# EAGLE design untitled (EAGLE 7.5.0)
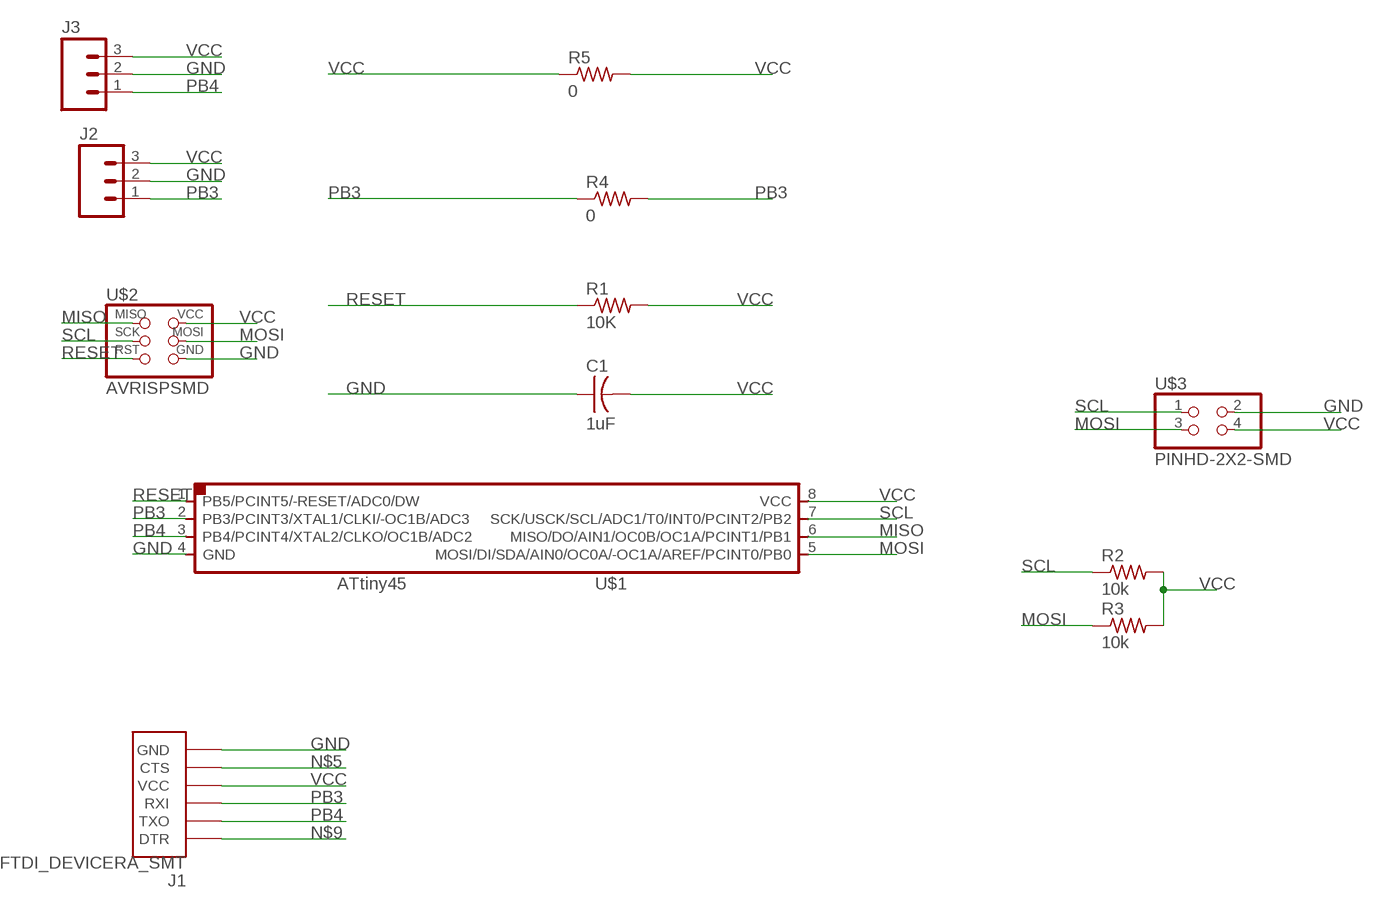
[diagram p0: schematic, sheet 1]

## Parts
C1  1uF  CAP-US1206  [C1206]
J1  FTDI_DEVICERA_SMT  [FTDI_DEVICE_RA_SMT]
J2  M03SMD_RA_MALE  [1X03_SMD_RA_MALE]
J3  M03SMD_RA_MALE  [1X03_SMD_RA_MALE]
R1  10K  RES-US1206FAB  [R1206FAB]
R2  10k  RES-US1206FAB  [R1206FAB]
R3  10k  RES-US1206FAB  [R1206FAB]
R4  0  RES-US1206FAB  [R1206FAB]
R5  0  RES-US1206FAB  [R1206FAB]
U$1  ATTINY45SI  [SOIC8]
U$2  AVRISPSMD  [2X03SMD]
U$3  PINHD-2X2-SMD  [2X02SMD]

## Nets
GND: C1.1 J1.6(GND) J2.2 J3.2 U$1.4(GND) U$2.6(GND) U$3.2
MISO: U$1.6(MISO/DO/AIN1/OC0B/OC1A/PCINT1/PB1) U$2.1(MISO)
MOSI: R3.1 U$1.5(MOSI/DI/SDA/AIN0/OC0A/-OC1A/AREF/PCINT0/PB0) U$2.4(MOSI) U$3.3
N$5: J1.5(CTS)
N$9: J1.1(DTR)
PB3: J1.3(RXI) J2.1 R4.1 R4.2 U$1.2(PB3/PCINT3/XTAL1/CLKI/-OC1B/ADC3)
PB4: J1.2(TXO) J3.1 U$1.3(PB4/PCINT4/XTAL2/CLKO/OC1B/ADC2)
RESET: R1.1 U$1.1(PB5/PCINT5/-RESET/ADC0/DW) U$2.5(RST)
SCL: R2.1 U$1.7(SCK/USCK/SCL/ADC1/T0/INT0/PCINT2/PB2) U$2.3(SCK) U$3.1
VCC: C1.2 J1.4(VCC) J2.3 J3.3 R1.2 R2.2 R3.2 R5.1 R5.2 U$1.8(VCC) U$2.2(VCC) U$3.4

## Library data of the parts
C1 = fab:CAP-US
J1 = SparkFun-Connectors:FTDI_DEVICE: Connector which mates to FTDI basic or FTDI cable.; PROD_ID: CONN-08971
J2 J3 = SparkFun-Connectors:M03: Header 3 Standard 3-pin 0.1" header. Use with straight break away headers (SKU : PRT-00116), right angle break away headers (PRT-00553), swiss pins (PRT-00743), machine pins (PRT-00117), and female headers (PRT-00115). Molex polarized connector foot print use with SKU : PRT-08232 with associated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; PROD_ID: CONN-10925
R1-R5 = fab:RES-US: Resistor (US Symbol)
U$1 = fab:ATTINY45
U$2 = fab:AVRISP
U$3 = fab:PINHD-2X2-SMD

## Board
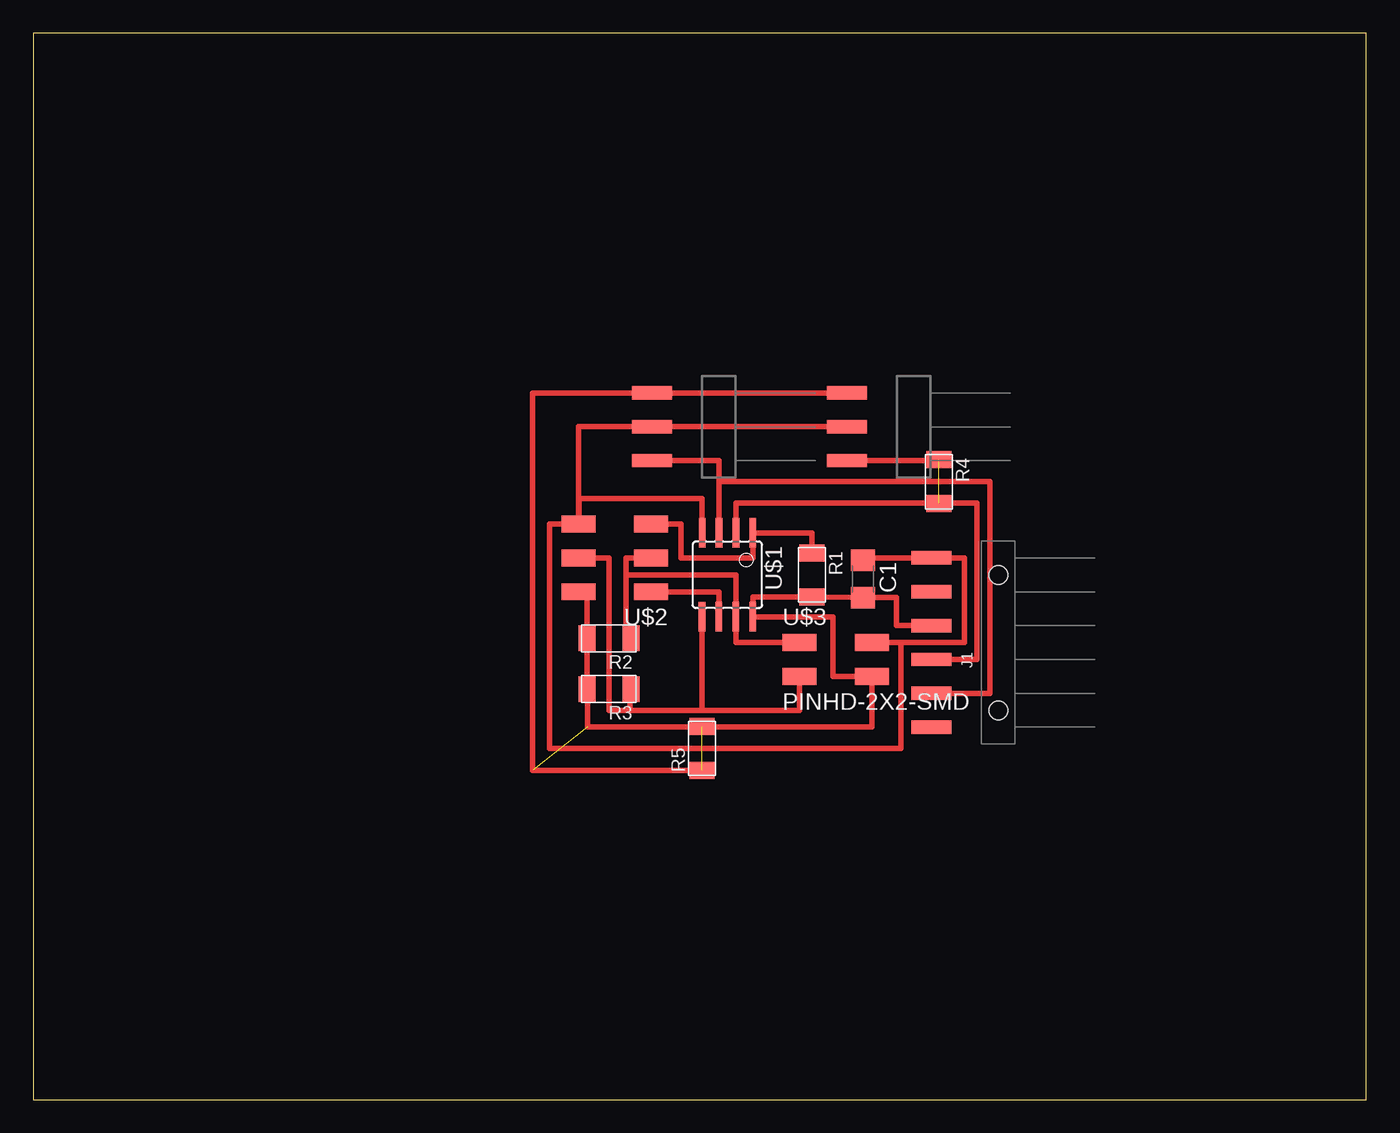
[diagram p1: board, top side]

Size 100 x 80 mm. Coordinates in mm from the lower left corner, seen from the top.
Outline: 0,0 100,0 100,80 0,80 0,0
Copper layers (1*16): Top 0.035mm / dielectric 1.5mm / Bottom 0.035mm
Design rules "default": minimum track width 10mil, minimum drill 24mil, track to track 8mil, track to pad 8mil, pad to pad 8mil, via to via 8mil, smd to smd 8mil, copper to edge 40mil, drill to drill 8mil, minimum pad ring 10mil, minimum via ring 8mil, stop-mask expansion 4mil, vias tented up to drill 0mil, thermal gap 10mil

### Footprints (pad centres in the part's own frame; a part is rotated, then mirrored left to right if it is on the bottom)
C1206 = smd 1.6 x 1.8: 1 -1.4,0; 2 1.4,0
FTDI_DEVICE_RA_SMT = smd 1 x 3: 1 -6.35,5; 2 -3.81,5; 3 -1.27,5; 4 1.27,5; 5 3.81,5; 6 6.35,5 | hole 1.4: -5.08,0; 5.08,0
1X03_SMD_RA_MALE = smd 1 x 3: 1 -2.54,5; 2 0,5; 3 2.54,5
R1206FAB = smd 1.27 x 1.905: 1 -1.651,0; 2 1.651,0
SOIC8 = smd 0.5 x 2.2: 1 -1.905,-3.154; 2 -0.645,-3.154; 3 0.625,-3.154; 4 1.895,-3.154; 5 1.905,3.154; 6 0.635,3.154; 7 -0.635,3.154; 8 -1.905,3.154
2X03SMD = smd 2.54 x 1.27: 1 -2.54,2.54; 2 2.92,2.54; 3 -2.54,0; 4 2.92,0; 5 -2.54,-2.54; 6 2.92,-2.54
2X02SMD = smd 2.54 x 1.27: 1 -2.54,1.27; 2 2.92,1.27; 3 -2.54,-1.27; 4 2.92,-1.27

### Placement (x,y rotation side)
C1  62.23,39.05 270 top
J1  72.39,34.29 90 top
J2  66.04,50.48 90 top
J3  51.44,50.48 90 top
R1  58.42,39.37 270 top
R2  43.18,34.61 180 top
R3  43.18,30.8 180 top
R4  67.94,46.35 270 top
R5  50.16,26.35 90 top
U$1  52.07,39.37 180 top
U$2  43.81,40.64 180 top
U$3  60.01,33.02 0 top

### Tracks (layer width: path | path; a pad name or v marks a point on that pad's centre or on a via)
GND
  Top 0.406: 65.09,34.29 69.85,34.29 69.85,40.64 J1.6 62.23,40.64 C1.1 | 62.61,34.29 U$3.2 65.09,34.29 | U$2.6 40.96,43.18 40.96,45.09 50.16,45.09 | 50.16,45.09 50.17,45.09 U$1.4 | U$1.4 50.16,42.23 | U$1.4 50.16,45.09 | U$2.6 38.73,43.18 38.73,26.35 65.09,26.35 65.09,34.29 | U$2.6 40.9,50.48 J3.2 J2.2
MISO
  Top 0.406: U$1.6 51.44,38.1 U$2.1
MOSI
  Top 0.406: 50.16,29.21 44.77,29.21 | 44.77,29.21 43.18,29.21 43.18,40.64 U$2.4 | U$1.5 50.16,29.21 | U$3.3 57.47,29.21 50.16,29.21 | R3.1 44.77,30.8 44.77,29.21
PB3  (1 unrouted)
  Top 0.406: J1.3 70.8,33.02 70.8,44.77 67.94,44.77 | 67.94,44.77 52.72,44.77 U$1.2 | J2.1 68.26,47.94 R4.1 | R4.2 67.94,44.77
PB4
  Top 0.406: J1.2 71.75,30.48 71.75,46.35 51.45,46.35 U$1.3 51.44,42.52 51.44,47.94 J3.1
RESET
  Top 0.406: R1.1 58.42,42.52 U$1.1 53.98,40.64 48.58,40.64 48.58,43.18 U$2.5
SCL
  Top 0.406: 58.1,34.29 U$3.1 52.7,34.29 U$1.7 52.7,39.37 44.45,39.37 | R2.1 44.45,34.92 44.45,39.37 | U$2.3 44.45,40.64 44.45,39.37
VCC  (2 unrouted)
  Top 0.406: J1.4 64.77,35.56 64.77,37.65 C1.2 R1.2 53.98,37.72 U$1.8 60.01,36.22 60.01,31.75 U$3.4 62.93,27.94 41.59,27.94 41.59,30.8 R3.2 R2.2 41.53,38.1 U$2.2 | J2.3 J3.3 37.47,53.02 37.47,24.7 R5.1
